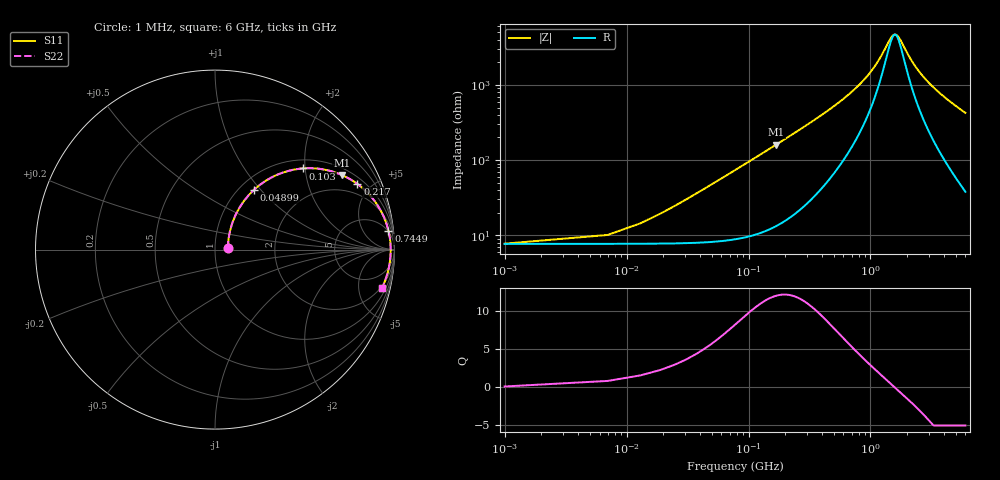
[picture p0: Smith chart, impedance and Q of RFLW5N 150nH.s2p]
!Vishay Electro-Films
!RFLW5N1500A - 150 nH Spiral Inductor on Quartz
!Measured in series configuration
!May 2011
# GHz S MA R 50
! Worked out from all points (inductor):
!   1001 points, 1 MHz to 6 GHz, reference 50 ohm
!   read as one part in series: L = 149 nH near 31 MHz
!   highest Q = 12.1 at 169 MHz (marker M1), where L = 151 nH
!   self-resonance near 1.588 GHz
!   S11 on the Smith chart (normalised r, x): 1 MHz: 1.15, +0.02; 48.99 MHz: 1.16, +0.92; 103 MHz: 1.19, +1.94; 217 MHz: 1.34, +4.15; 744.9 MHz: 5, +17; 6 GHz: 1.76, -8.45
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0.001  0.07192 6.5  0.9286 -0.5  0.9286 -0.5  0.07192 6.5
0.024996  0.2243 59.3  0.9063 -12.3  0.9063 -12.3  0.2243 59.3
0.048992  0.3979 56.9  0.8507 -23.1  0.8507 -23.1  0.3979 56.9
0.072988  0.5385 50.5  0.7776 -32.3  0.7776 -32.3  0.5385 50.5
0.102983  0.666 42.8  0.6824 -41.5  0.6824 -41.5  0.666 42.8
0.132978  0.7521 36.4  0.596 -48.5  0.596 -48.5  0.7521 36.4
0.168972  0.8195 30.5  0.5093 -54.8  0.5093 -54.8  0.8195 30.5
0.216964  0.8737 24.8  0.4201 -60.5  0.4201 -60.5  0.8737 24.8
0.288952  0.9168 19.0  0.3265 -66.0  0.3265 -66.0  0.9168 19.0
0.390935  0.9453 13.9  0.2422 -70.1  0.2422 -70.1  0.9453 13.9
0.546909  0.9633 9.5  0.1663 -72.5  0.1663 -72.5  0.9633 9.5
0.744876  0.9722 6.2  0.1102 -72.3  0.1102 -72.3  0.9722 6.2
1.00283  0.9767 3.6  0.06568 -67.4  0.06568 -67.4  0.9767 3.6
1.42276  0.9789 0.8  0.02547 -33.5  0.02547 -33.5  0.9789 0.8
1.55474  0.979 0.2  0.02114 -7.3  0.02114 -7.3  0.979 0.2
1.69272  0.9791 -0.5  0.02253 21.4  0.02253 21.4  0.9791 -0.5
2.00467  0.9787 -1.8  0.03717 54.2  0.03717 54.2  0.9787 -1.8
2.43659  0.9776 -3.3  0.06132 66.9  0.06132 66.9  0.9776 -3.3
3.0005  0.9754 -5.1  0.09108 71.8  0.09108 71.8  0.9754 -5.1
4.00233  0.97 -7.9  0.1392 73.6  0.1392 73.6  0.97 -7.9
5.00417  0.9629 -10.5  0.1836 73.1  0.1836 73.1  0.9629 -10.5
6  0.9544 -13.0  0.2251 71.9  0.2251 71.9  0.9544 -13.0
